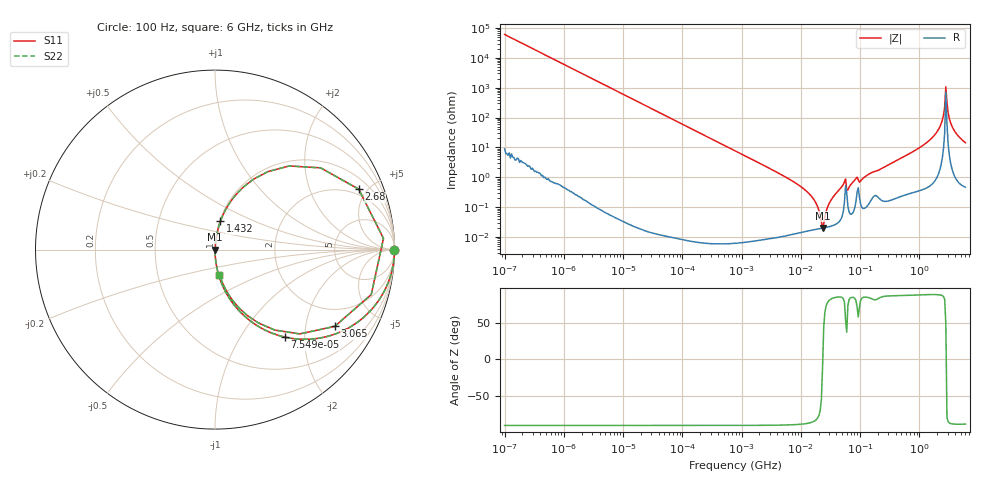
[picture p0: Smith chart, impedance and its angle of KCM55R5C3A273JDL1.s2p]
!Murata Part Number: KCM55R5C3A273JDL1
!These Parameters are Measured in Series Mode Connection
!Data Generated on Mar 13, 2026
!  o--ll--o
!Port1  Port2
!  o------o
!Operation Temp=25[degC], DC Bias Voltage=0[V]
!Freq. Start=100[Hz] Stop=6[GHz] 401[Steps]
# Hz S RI R 50
!Freq.(Hz) S11(Real) S11(Imag) S21(Real) S21(Imag) S12(Real) S12(Imag) S22(Real) S22(Imag)
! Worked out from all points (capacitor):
!   401 points, 100 Hz to 6 GHz, reference 50 ohm
!   read as one part in series: C = 26.4 nF near 109 Hz
!   lowest |Z| = 20.2 mohm at 23.28 MHz (marker M1)
!   series resonance near 23.46 MHz, so ESL is about 1.7 nH
!   S11 on the Smith chart (normalised r, x): 100 Hz: open; 75.5 kHz: 1.00, -1.60; 1.432 GHz: 1.01, +0.33; 2.68 GHz: 1.60, +4.40; 3.065 GHz: 1.27, -2.91; 6 GHz: 1.01, -0.29
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100  1 -0.00166  3e-06 0.00166  3e-06 0.00166  1 -0.00166
2008  0.9989 -0.0333  0.00111 0.0333  0.00111 0.0333  0.9989 -0.0333
14402  0.946 -0.2261  0.054 0.2261  0.054 0.2261  0.946 -0.2261
40335  0.6906 -0.4622  0.3094 0.4622  0.3094 0.4622  0.6906 -0.4622
75495  0.3893 -0.4875  0.6107 0.4875  0.6107 0.4875  0.3893 -0.4875
193316  0.0886 -0.2841  0.9114 0.2841  0.9114 0.2841  0.0886 -0.2841
774597  0.00606 -0.0772  0.9939 0.0772  0.9939 0.0772  0.00606 -0.0772
6948629  0.000183 -0.00788  0.9998 0.00788  0.9998 0.00788  0.000183 -0.00788
1.555665e7  0.000176 -0.00216  0.9998 0.00216  0.9998 0.00216  0.000176 -0.00216
2.327686e7  0.000198 -3.98e-05  0.9998 3.98e-05  0.9998 3.98e-05  0.000198 -3.98e-05
3.184506e7  0.000233 0.00163  0.9998 -0.00163  0.9998 -0.00163  0.000233 0.00163
5.211241e7  0.000754 0.00573  0.9992 -0.00573  0.9992 -0.00573  0.000754 0.00573
6.518806e7  0.000722 0.0046  0.9993 -0.0046  0.9993 -0.0046  0.000722 0.0046
3.124326e8  0.00239 0.0272  0.9976 -0.0272  0.9976 -0.0272  0.00239 0.0272
1.431855e9  0.0303 0.1575  0.9697 -0.1575  0.9697 -0.1575  0.0303 0.1575
2.142435e9  0.1614 0.3515  0.8386 -0.3515  0.8386 -0.3515  0.1614 0.3515
2.450438e9  0.4138 0.466  0.5862 -0.466  0.5862 -0.466  0.4138 0.466
2.679998e9  0.8009 0.3365  0.1991 -0.3365  0.1991 -0.3365  0.8009 0.3365
3.065283e9  0.6672 -0.4278  0.3328 0.4278  0.3328 0.4278  0.6672 -0.4278
3.352442e9  0.3327 -0.4483  0.6673 0.4483  0.6673 0.4483  0.3327 -0.4483
3.8344e9  0.1367 -0.3279  0.8633 0.3279  0.8633 0.3279  0.1367 -0.3279
6e9  0.0247 -0.14  0.9753 0.14  0.9753 0.14  0.0247 -0.14
